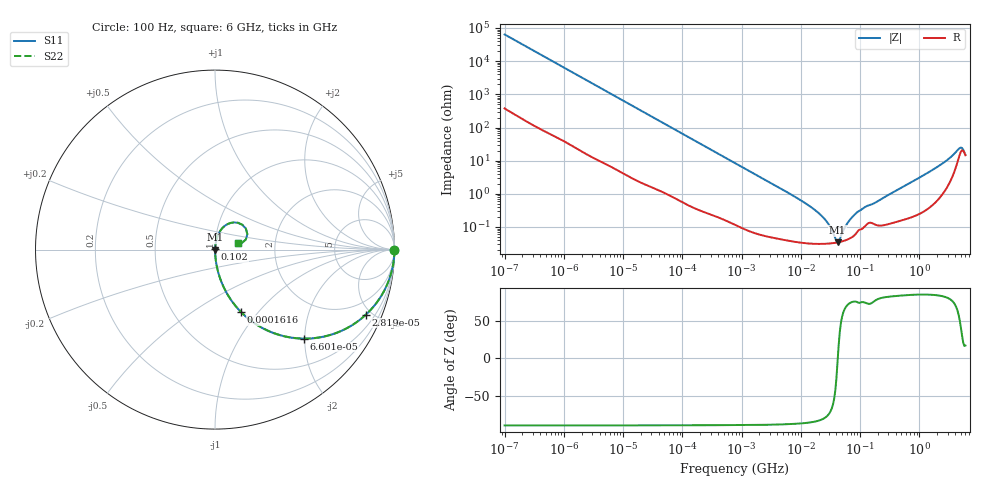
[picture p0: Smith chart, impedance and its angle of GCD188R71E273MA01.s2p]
!Murata Part Number: GCD188R71E273MA01
!These Parameters are Measured in Series Mode Connection
!Data Generated on Mar 13, 2026
!  o--ll--o
!Port1  Port2
!  o------o
!Operation Temp=25[degC], DC Bias Voltage=0[V]
!Freq. Start=100[Hz] Stop=6[GHz] 401[Steps]
# Hz S RI R 50
!Freq.(Hz) S11(Real) S11(Imag) S21(Real) S21(Imag) S12(Real) S12(Imag) S22(Real) S22(Imag)
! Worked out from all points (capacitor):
!   401 points, 100 Hz to 6 GHz, reference 50 ohm
!   read as one part in series: C = 24.9 nF near 109 Hz
!   lowest |Z| = 34.5 mohm at 41.66 MHz (marker M1)
!   series resonance near 42.08 MHz, so ESL is about 570 pH
!   S11 on the Smith chart (normalised r, x): 100 Hz: open; 28.19 kHz: 1.03, -4.62; 66 kHz: 1.02, -1.98; 161.6 kHz: 1.01, -0.81; 102 MHz: 1.00, +0.01; 6 GHz: 1.29, +0.09
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100  1 -0.00157  1.17e-05 0.00157  1.17e-05 0.00157  1 -0.00157
2008  0.9988 -0.0311  0.00115 0.0311  0.00115 0.0311  0.9988 -0.0311
8801  0.9811 -0.133  0.0189 0.133  0.0189 0.133  0.9811 -0.133
28191  0.8404 -0.3626  0.1596 0.3626  0.1596 0.3626  0.8404 -0.3626
40335  0.7219 -0.4442  0.2781 0.4442  0.2781 0.4442  0.7219 -0.4442
66005  0.4956 -0.4958  0.5044 0.4958  0.5044 0.4958  0.4956 -0.4958
161617  0.1441 -0.3467  0.8559 0.3467  0.8559 0.3467  0.1441 -0.3467
302498  0.0474 -0.2071  0.9526 0.2071  0.9526 0.2071  0.0474 -0.2071
774597  0.00843 -0.0849  0.9916 0.0849  0.9916 0.0849  0.00843 -0.0849
1.555665e7  0.000328 -0.00375  0.9997 0.00375  0.9997 0.00375  0.000328 -0.00375
2.662322e7  0.000316 -0.00153  0.9997 0.00153  0.9997 0.00153  0.000316 -0.00153
3.80911e7  0.000335 -0.000322  0.9997 0.000322  0.9997 0.000322  0.000335 -0.000322
4.165952e7  0.000344 -3.21e-05  0.9997 3.21e-05  0.9997 3.21e-05  0.000344 -3.21e-05
4.556224e7  0.000356 0.000258  0.9996 -0.000258  0.9996 -0.000258  0.000356 0.000258
5.449875e7  0.000389 0.000847  0.9996 -0.000847  0.9996 -0.000847  0.000389 0.000847
6.518806e7  0.000443 0.00147  0.9996 -0.00147  0.9996 -0.00147  0.000443 0.00147
1.020051e8  0.000852 0.00311  0.9991 -0.00311  0.9991 -0.00311  0.000852 0.00311
3.124326e8  0.00133 0.00956  0.9987 -0.00956  0.9987 -0.00956  0.00133 0.00956
2.562649e9  0.0177 0.0835  0.9823 -0.0835  0.9823 -0.0835  0.0177 0.0835
4.586474e9  0.1281 0.1493  0.8719 -0.1493  0.8719 -0.1493  0.1281 0.1493
5.245841e9  0.1803 0.0862  0.8197 -0.0862  0.8197 -0.0862  0.1803 0.0862
6e9  0.1288 0.0346  0.8712 -0.0346  0.8712 -0.0346  0.1288 0.0346
